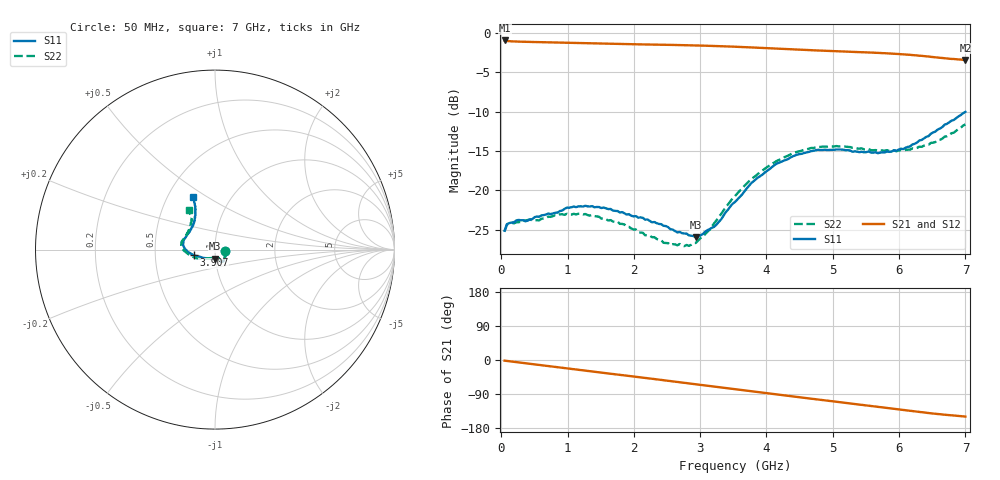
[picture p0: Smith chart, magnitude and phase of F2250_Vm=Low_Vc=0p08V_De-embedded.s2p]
! Integrated Device Technology
! Corporate Headquarters
! 6024 Silver Creek Valley Road
! San Jose, CA 95138  USA
! Phone:  1-408-284-8200
! Toll Free:  1-800-223-1366
! Webpage:  http://www.idt.com/
! Timing and RF Division
! 515 Groton Road, Suite 102
! Westford, MA 01886-6024
! Device:  F2250
! Description: Voltage Variable RF Attenuator
! Frequency:  50.0 -  6000.00 MHz
! Package:  3x3 mm Thin QFN Plastic Package: 16 pin
! Ports:  2 RF, 3 DC
!  Pin  1  = GND
!  Pin  2  = NC
!  Pin  3  = RF1  = Port 1
!  Pin  4  = NC
!  Pin  5  = GND
!  Pin  6  = GND
!  Pin  7  = GND
!  Pin  8  = GND
!  Pin  9  = NC
!  Pin 10  = RF2  = Port 2
!  Pin 11  = NC
!  Pin 12  = GND
!  Pin 13  = GND
!  Pin 14  = VCNTRL
!  Pin 15  = VDD
!  Pin 16  = VMODE
! Vcntrl:  0.080 Volts
! Vmode:  +0.000 Volts
! Vdd:  +3.30  Volts
! Current:  1.105 mA
! Data:  The device was measured on a the F2250 evaluation board which has
!  individual transmission lines to the RF pins.  Data was collected
!  using a calibrated network analyzer.  The evaluation board was
!  de-embedded using a TRL calibration technique.
!  The reference plane is the edge of the package pin.
! Misc:  SN 10
!  Action Tracker AT0258
! Date Measured:  2014-11-26
! Date:  2015-10-15  MJV
! Note:
!  Integrated Device Technology supplies this data as a sample of measured
!  data at the package pin for this product.  Your particular data for this
!  product may vary.
!  Data was taken at 25 degrees C.
!  Integrated Device Technology reserves the right to change this data at anytime.
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# GHz S dB R 50
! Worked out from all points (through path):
!   201 points, 50 MHz to 7 GHz, reference 50 ohm
!   highest |S21| = -0.93 dB at 50 MHz (marker M1); lowest = -3.4 dB at 7 GHz (marker M2)
!   group delay of S21, straight-line fit = 59.9 ps
!   lowest |S11| = -26.0 dB at 2.934 GHz (marker M3), VSWR 1.11, Z = 49.5 - j4.99 ohm
!   |S11| at or under -10 dB: start of sweep to end of sweep
!   |S22| runs from -27.1 to -11.6 dB; largest |S21 - S12| = 0.0003
!   S11 on the Smith chart (normalised r, x): 50 MHz: 1.12, -0.02; 3.907 GHz: 0.79, -0.05; 7 GHz: 0.67, +0.43
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0.05  -25.12 -9.8  -0.93 -1.8  -0.93 -1.8  -25.22 -10.1
0.08475  -24.29 -9.7  -0.99 -2.5  -0.99 -2.5  -24.35 -9.4
0.15425  -24.08 -11.9  -1.04 -4.0  -1.04 -3.9  -24.10 -11.0
0.57125  -23.35 -30.1  -1.14 -13.1  -1.14 -13.1  -23.81 -30.4
0.884  -22.62 -45.9  -1.20 -19.9  -1.20 -19.9  -23.05 -46.8
1.2315  -22.06 -56.1  -1.28 -27.4  -1.28 -27.4  -23.05 -59.7
1.75275  -22.62 -62.8  -1.37 -38.4  -1.37 -38.4  -23.95 -66.6
2.37825  -24.26 -63.6  -1.46 -51.8  -1.46 -51.8  -26.29 -67.8
2.552  -24.94 -67.8  -1.49 -55.6  -1.49 -55.6  -26.95 -73.3
2.83  -25.72 -83.3  -1.54 -61.7  -1.54 -61.7  -27.06 -92.6
2.93425  -25.97 -92.4  -1.56 -64.0  -1.56 -64.0  -26.68 -101.6
3.21225  -24.62 -122.1  -1.63 -70.1  -1.63 -70.1  -24.17 -127.6
3.525  -21.47 -148.3  -1.72 -77.0  -1.72 -77.0  -20.72 -146.4
3.76825  -19.09 -161.3  -1.81 -82.4  -1.81 -82.4  -18.56 -156.7
3.90725  -18.18 -165.6  -1.87 -85.4  -1.87 -85.4  -17.67 -162.8
4.1505  -16.61 -173.7  -1.97 -90.7  -1.96 -90.7  -16.27 -171.4
4.7065  -14.96 172.3  -2.18 -102.7  -2.18 -102.7  -14.60 175.7
5.15825  -14.82 161.5  -2.33 -112.5  -2.33 -112.5  -14.37 166.6
5.85325  -15.10 138.5  -2.58 -127.4  -2.58 -127.4  -15.00 151.6
6.166  -14.40 127.6  -2.75 -134.2  -2.76 -134.2  -14.81 142.7
6.444  -13.10 119.3  -2.96 -140.0  -2.96 -140.0  -14.19 133.4
7  -10.01 113.1  -3.41 -149.2  -3.41 -149.2  -11.60 123.9
